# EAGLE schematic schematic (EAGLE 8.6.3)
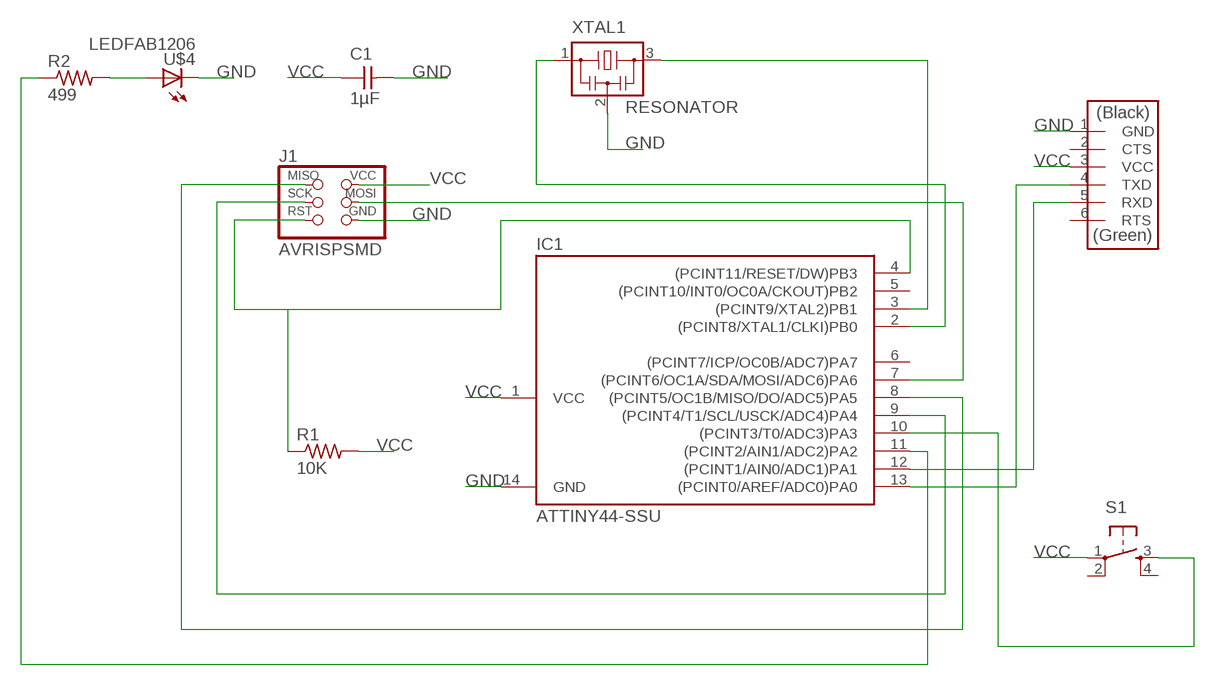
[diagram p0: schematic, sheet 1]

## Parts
C1  1µF  CAP-UNPOLARIZEDFAB  [C1206FAB]
IC1  ATTINY44-SSU  [SOIC14]
J1  AVRISPSMD  [2X03SMD]
R1  10K  RES-US1206FAB  [R1206FAB]
R2  499  RES-US1206FAB  [R1206FAB]
S1  6MM_SWITCH6MM_SWITCH  [6MM_SWITCH]
U$3  FTDI-SMD-HEADER  [1X06SMD]
U$4  LEDFAB1206  [LED1206FAB]
XTAL1  RESONATOR  [EFOBM]

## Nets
GND: C1.2 IC1.14(GND) J1.6(GND) U$3.1(GND) U$4.2(C) XTAL1.2
N$1: IC1.8((PCINT5/OC1B/MISO/DO/ADC5)PA5) J1.1(MISO)
N$2: IC1.7((PCINT6/OC1A/SDA/MOSI/ADC6)PA6) J1.4(MOSI)
N$3: IC1.9((PCINT4/T1/SCL/USCK/ADC4)PA4) J1.3(SCK)
N$4: IC1.12((PCINT1/AIN0/ADC1)PA1) U$3.5(RXD)
N$5: IC1.13((PCINT0/AREF/ADC0)PA0) U$3.4(TXD)
N$6: IC1.3((PCINT9/XTAL2)PB1) XTAL1.3
N$7: IC1.2((PCINT8/XTAL1/CLKI)PB0) XTAL1.1
N$8: IC1.4((PCINT11/RESET/DW)PB3) J1.5(RST) R1.1
N$9: R2.2 U$4.1(A)
N$10: IC1.11((PCINT2/AIN1/ADC2)PA2) R2.1
N$11: IC1.10((PCINT3/T0/ADC3)PA3) S1.3(S)
VCC: C1.1 IC1.1(VCC) J1.2(VCC) R1.2 S1.1(P) U$3.3(VCC)
Unconnected: IC1.5((PCINT10/INT0/OC0A/CKOUT)PB2) IC1.6((PCINT7/ICP/OC0B/ADC7)PA7) S1.2(P1) S1.4(S1) U$3.2(CTS) U$3.6(RTS)

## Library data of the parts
C1 = fab:CAP-UNPOLARIZED
IC1 = fab:ATTINY44
J1 = fab:AVRISP
R1 R2 = fab:RES-US: Resistor (US Symbol)
S1 = fab:6MM_SWITCH: OMRON SWITCH
U$3 = fab:FTDI-SMD-HEADER
U$4 = fab:LED: LED
XTAL1 = fab:RESONATOR

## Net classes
0 default: clearance 0.205 mm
